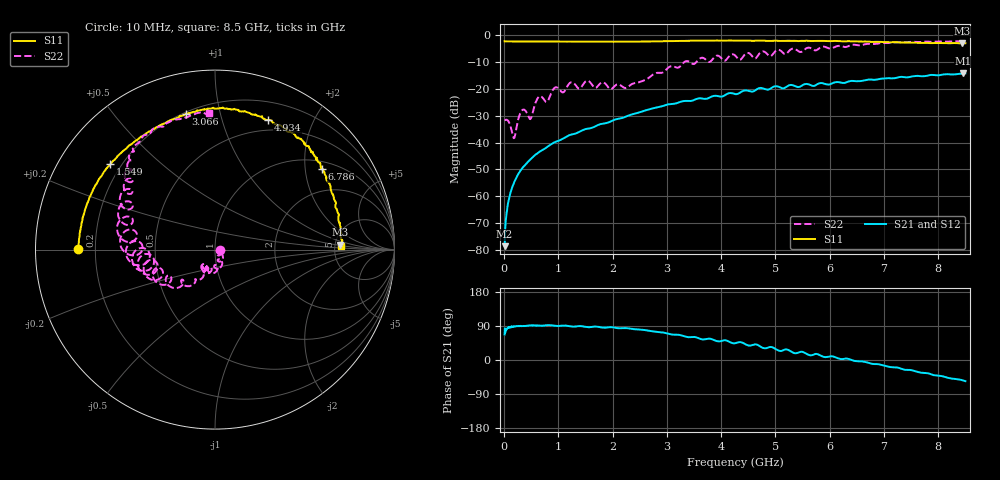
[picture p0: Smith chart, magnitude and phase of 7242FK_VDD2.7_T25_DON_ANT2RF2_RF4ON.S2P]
!Agilent Technologies,E5071C,MY46417908,A.11.23
!Date: Wed Dec 09 15:39:58 2020
!Data & Calibration Information:
!Freq	S11:SOLT2(ON)	S21:SOLT2(ON)	S12:SOLT2(ON)	S22:SOLT2(ON)
!PortZ  Port1:50+j0  Port2:50+j0
!Above PortZ is port z conversion or system Z0 setting when saving the data.
!When reading, reference impedance value at option line is always used.
# Hz S dB R 50
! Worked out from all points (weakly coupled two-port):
!   1601 points, 10 MHz to 8.5 GHz, reference 50 ohm
!   highest |S21| = -14.24 dB at 8.458 GHz (marker M1); lowest = -78.6 dB at 10 MHz (marker M2)
!   lowest |S11| = -3.1 dB at 8.442 GHz (marker M3), VSWR 5.61, Z = 277 + j29.7 ohm
!   |S11| at or under -10 dB: nowhere
!   |S22| runs from -38.4 to -2.3 dB; largest |S21 - S12| = 0.003
!   S11 on the Smith chart (normalised r, x): 10 MHz: 0.13, +0.00; 1.549 GHz: 0.16, +0.35; 3.066 GHz: 0.21, +0.79; 4.934 GHz: 0.38, +1.42; 6.786 GHz: 1.21, +2.45; 8.5 GHz: 5.71, +0.46
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1e7  -2.35 179.7  -78.57 67.4  -77.61 79.4  -31.74 -2.9
7.898125e7  -2.38 177.8  -62.00 87.1  -61.77 84.8  -32.03 -32.4
1.851062e8  -2.40 175.0  -54.88 88.7  -54.91 87.8  -38.35 -24.4
3.177625e8  -2.41 171.4  -49.99 89.5  -50.02 89.3  -28.37 -27.8
4.875625e8  -2.41 166.9  -46.22 91.1  -46.24 91.2  -31.20 -49.4
6.308312e8  -2.41 163.3  -43.78 90.8  -43.77 91.0  -23.16 -52.7
7.900188e8  -2.43 159.6  -41.73 91.8  -41.71 91.8  -24.86 -68.4
9.439e8  -2.43 155.7  -39.80 90.3  -39.78 90.3  -19.50 -77.4
1.426769e9  -2.45 143.9  -35.60 89.2  -35.60 89.2  -19.28 -99.9
1.548812e9  -2.47 140.8  -34.82 86.5  -34.83 86.5  -17.04 -115.5
1.676162e9  -2.49 137.7  -34.01 88.2  -34.03 88.2  -19.68 -118.3
2.243931e9  -2.49 122.5  -30.37 84.2  -30.37 84.2  -19.71 -119.0
2.843538e9  -2.35 106.8  -26.82 73.5  -26.83 73.6  -14.06 -123.4
3.0664e9  -2.24 102.2  -25.67 68.0  -25.68 68.0  -11.66 -129.9
4.255e9  -2.06 80.5  -21.95 44.1  -21.96 44.1  -7.58 -174.5
4.9342e9  -2.16 67.8  -19.59 34.0  -19.58 34.0  -7.55 -177.1
5.671769e9  -2.25 53.8  -18.84 12.6  -18.78 12.5  -5.07 151.1
6.786081e9  -2.55 37.1  -16.60 -10.3  -16.63 -10.1  -3.33 133.1
7.088538e9  -2.69 32.3  -16.04 -17.8  -16.10 -17.9  -2.98 129.6
8.441631e9  -3.13 2.3  -14.29 -53.3  -14.37 -53.4  -2.40 93.9
8.45755e9  -3.12 1.9  -14.24 -53.9  -14.33 -54.1  -2.39 93.4
8.5e9  -3.05 1.6  -14.24 -55.8  -14.35 -55.6  -2.35 92.5
